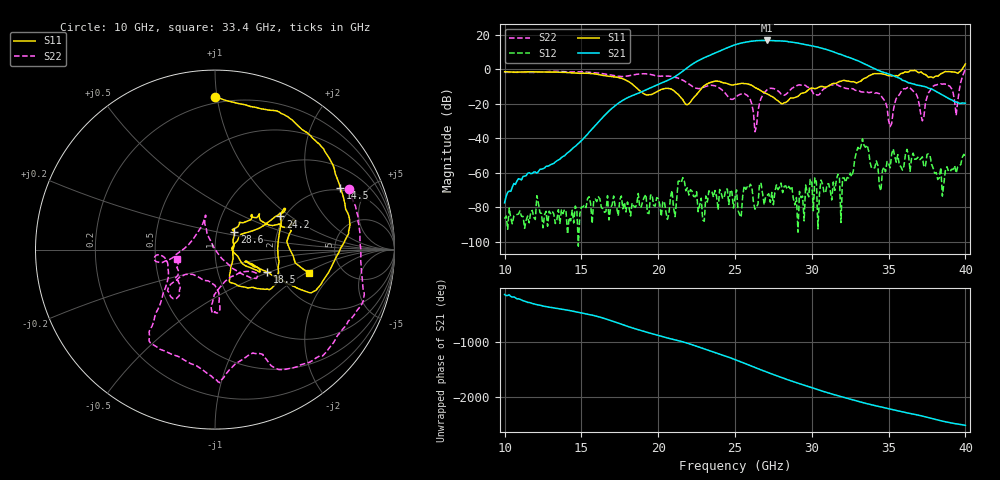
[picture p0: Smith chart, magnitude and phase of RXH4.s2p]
!Keysight Technologies,M9808A,MY58100618,A.14.70.03
!Date: Monday, February 27, 2023 13:43:34
!Correction: S11(Cdelta 2-Port  )
!S21(Cdelta 2-Port  )
!S12(Cdelta 2-Port  )
!S22(Cdelta 2-Port  )
!S2P File: Measurements: S11, S21, S12, S22:
# Hz S  RI  R 50
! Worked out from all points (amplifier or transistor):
!   301 points, 10 GHz to 40 GHz, reference 50 ohm
!   highest |S21| = 16.7 dB at 27.1 GHz (marker M1)
!   |S21| within 3 dB of that: 24.84 GHz to 29.95 GHz (5.107 GHz wide, 18.6 % of centre)
!   unconditionally stable (mu >= 1): start of sweep to 39.73 GHz
!   at 15 GHz: K = 68908.92, MAG = -32.2 dB, |S12| = -79.8 dB
!   at 25 GHz: K = 448.87, MAG = 14.9 dB, |S12| = -74.6 dB
!   at 40 GHz: K = 53.83, MSG = 15.8 dB, |S12| = -51.3 dB
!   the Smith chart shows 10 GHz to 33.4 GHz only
!   S11 on the Smith chart (normalised r, x): 10 GHz: 0.16, +0.98; 14.5 GHz: 1.91, +3.30; 18.5 GHz: 1.73, -0.48; 24.2 GHz: 1.90, +0.84; 28.6 GHz: 1.22, +0.24; 33.4 GHz: 2.92, -1.07
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1e10  -0.00253 0.85  -0.000121 -6.03e-05  4.31e-05 -1.77e-05  0.7448 0.3374
1.45e10  0.6991 0.3413  -0.000466 -0.00542  2.45e-05 2.5e-05  0.669 -0.5036
1.5e10  0.7384 0.2055  -0.00454 -0.0072  8.67e-05 5.38e-05  0.6108 -0.5801
1.85e10  0.2896 -0.1239  0.1208 -0.1411  -1.8e-05 9.78e-05  0.0569 -0.6986
2e10  0.2168 -0.0955  -0.358 -0.0657  -7.96e-05 0.000163  -0.1689 -0.6167
2.28e10  0.2464 0.1192  1.667 -1.049  6.26e-05 -0.000174  -0.2814 -0.0436
2.42e10  0.3646 0.1849  -3.508 -1.126  0.000104 0.000144  -0.2358 -0.0452
2.5e10  0.3567 -0.0669  -2.319 4.552  -4.04e-05 0.000181  -0.0754 0.1277
2.55e10  0.3365 -0.1961  2.658 5.229  -0.000211 -2.85e-05  -0.0538 0.1907
2.61e10  0.2603 -0.2196  6.501 -0.2793  -0.000168 0.000347  -0.0439 0.086
2.66e10  0.1468 -0.2062  3.629 -5.771  -0.000365 -0.00034  0.0707 -0.0788
2.71e10  0.0789 -0.1747  -2.409 -6.396  -0.000186 -0.000123  0.201 -0.1583
2.78e10  0.0956 -0.0754  -6.688 0.2092  -0.000324 3.17e-05  0.2008 -0.1212
2.86e10  0.1083 0.0971  -0.9243 6.12  7.02e-05 0.000334  -0.00424 -0.252
2.94e10  0.1357 0.1518  4.9 2.279  0.000201 6.14e-05  -0.00387 -0.3494
3e10  0.2057 0.1953  4.181 -2.294  0.000226 -0.000503  0.0212 -0.2402
3.06e10  0.2485 0.1987  0.5893 -4.094  -0.000613 8.42e-05  -0.1641 -0.1381
3.14e10  0.3603 0.1435  -2.766 -1.655  -0.00042 -0.000336  -0.2523 -0.2491
3.24e10  0.4297 0.1492  -1.487 1.638  -0.00027 0.000656  -0.2051 -0.1769
3.34e10  0.5247 -0.1293  0.7931 1.218  -0.00238 -0.00572  -0.2121 -0.0504
3.5e10  0.6486 0.00403  0.508 -0.5255  0.00103 -0.00158  -0.0315 -0.00799
4e10  1.292 -0.6123  0.1014 0.0228  -0.00273 -0.000245  0.4799 -0.894
